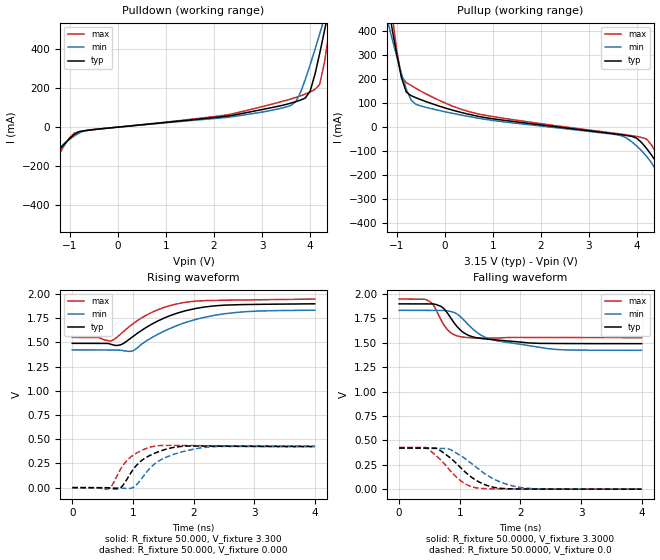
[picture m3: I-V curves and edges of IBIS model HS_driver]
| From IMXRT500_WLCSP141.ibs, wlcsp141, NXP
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[Model] HS_driver
|   Model HS_driver
| Library cells for typ/min/max conditions are connected as defined below:
|  pad_usbdp - External Pad
|  usb2_tx_d_data_dp - Core Input
|  gnda - gnda
|  pad_usb_vss - pad_usb_vss
|  usb2_reg_tx_fs_hiz - gnda
|  usb2_reg_tx_hs_term - vddd
|  usb2_reg_tx_hs_xcvr - vddd
|  usb2_reg_tx_ls_en - gnda
|  usbphy_d2a_txhsactive - vddd
|  vddb - vddb
|  vddd - vddd
| All other pins connected to ground
Model_type Output
Polarity   Non-Inverting
Enable   Active-High
C_comp   2.8431pF   2.6338pF   3.0727pF
[Temperature Range]   27.0000   0.1250k   -40.0000
[Voltage Range]   3.1500V   3.0000V   3.3000V
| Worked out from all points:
|   slope of the pulldown table from 0 to 0.472 V, typ, clamps not added: 41.5 ohm
|   slope of the pullup table from 0 to 0.472 V, typ, clamps not added: 18.7 ohm
|   rising waveform, R_fixture 50.000, V_fixture 3.300: 20-80 % time 788ps typ, 925ps min, 673ps max; typ from 1.49 V to 1.9 V
|   rising waveform, R_fixture 50.000, V_fixture 0.000: 20-80 % time 403ps typ, 514ps min, 316ps max; typ from 0 V to 0.424 V
|   falling waveform, R_fixture 50.0000, V_fixture 3.3000: 20-80 % time 376ps typ, 729ps min, 219ps max; typ from 1.9 V to 1.49 V
|   falling waveform, R_fixture 50.0000, V_fixture 0.0: 20-80 % time 478ps typ, 592ps min, 401ps max; typ from 0.422 V to 0 V
[Pulldown]
|Voltage   I(typ)   I(min)   I(max)
-3.3V     -1.789A    -1.328A    -2.415A
-2.1V     -625.7mA   -518.6mA   -789mA
-1.9V     -460.2mA   -400.2mA   -566.6mA
-1.4V     -174.1mA   -160.8mA   -216.9mA
-800mV    -22.89mA   -29.67mA   -23.37mA
3.6V      122.9mA    110.8mA    144.1mA
4V        183mA      317.7mA    180.5mA
4.2V      376.9mA    477.2mA    219mA
4.3V      493.6mA    559.9mA    332.1mA
4.4V      614.7mA    643.7mA    494.7mA
4.5V      738.7mA    728.1mA    671.8mA
6.6V      3.53A      2.592A     4.822A
[Pullup]
|Voltage   I(typ)   I(min)   I(max)
-3.3V     3.3A       2.299A     4.797A
-1.2V     532mA      451.2mA    654.1mA
-1.1V     415.8mA    372.2mA    481.1mA
-900mV    206.9mA    223.2mA    210.7mA
-700mV    130.9mA    112.5mA    173.3mA
700mV     45.05mA    37.34mA    54.91mA
3.9V      -38.79mA   -62.16mA   -35.71mA
4.3V      -115.3mA   -147.1mA   -73.13mA
4.6V      -211.6mA   -260.7mA   -191.1mA
4.9V      -368.9mA   -418mA     -342.3mA
5V        -440.4mA   -476.1mA   -413.1mA
6.6V      -1.963A    -1.562A    -2.435A
[Ramp]
| variable   typ   min   max
dV/dt_r  0.2425/0.3998n   0.2407/0.5102n   0.2458/0.3124n
dV/dt_f  0.2330/0.3629n   0.2298/0.6151n   0.2278/0.2332n
R_load = 45.0000
[Rising Waveform]
R_fixture = 50.000
V_fixture = 3.300
V_fixture_min = 3.000
V_fixture_max = 3.600
|  time   V(typ)   V(min)   V(max)
0s        1.489V     1.421V     1.55V
423.1ps   1.489V     1.421V     1.55V
635.7ps   1.48V      1.421V     1.514V
795.1ps   1.474V     1.417V     1.584V
989.5ps   1.554V     1.41V      1.686V
1.408ns   1.719V     1.581V     1.835V
1.906ns   1.831V     1.712V     1.917V
2.327ns   1.875V     1.776V     1.932V
2.7ns     1.887V     1.808V     1.936V
4ns       1.897V     1.831V     1.946V
[Rising Waveform]
R_fixture = 50.000
V_fixture = 0.000
V_fixture_min = 0.000
V_fixture_max = 0.000
|  time   V(typ)   V(min)   V(max)
0s        86.47nV    2.71uV     53.59nV
593.9ps   -1.371mV   1.709uV    -11.79mV
661ps     -10.2mV    -1.193uV   29.57mV
778.4ps   -6.653mV   -1.53mV    170.1mV
1.026ns   205.5mV    10.32mV    343.6mV
1.178ns   295.4mV    122.6mV    393.9mV
1.393ns   363.7mV    260.8mV    431.3mV
1.77ns    424.3mV    362.1mV    434.8mV
2.208ns   428.6mV    416.8mV    432.5mV
4ns       424.4mV    422.1mV    429.5mV
[Falling Waveform]
R_fixture= 50.0000
V_fixture= 3.3000
V_fixture_min= 3.0000
V_fixture_max= 3.6000
|time   V(typ)   V(min)   V(max)
0s        1.897V     1.831V     1.946V
504ps     1.897V     1.831V     1.921V
571.5ps   1.896V     1.831V     1.878V
686ps     1.872V     1.831V     1.738V
797.4ps   1.802V     1.826V     1.633V
1.027ns   1.62V      1.758V     1.559V
1.329ns   1.545V     1.585V     1.547V
1.664ns   1.526V     1.514V     1.549V
2.591ns   1.491V     1.431V     1.552V
4ns       1.49V      1.422V     1.551V
[Falling Waveform]
R_fixture= 50.0000
V_fixture= 0.0
V_fixture_min= 0.0
V_fixture_max= 0.0
|time   V(typ)   V(min)   V(max)
0s        421.7mV    418.5mV    427.2mV
441.6ps   421.8mV    418.5mV    426.2mV
625.8ps   415.8mV    418.5mV    335.7mV
805.8ps   339.1mV    414.1mV    216.4mV
994.4ps   232.6mV    351.5mV    95.97mV
1.262ns   93.77mV    228.8mV    14.73mV
1.448ns   38.4mV     144.5mV    4.904mV
1.624ns   12.57mV    85.57mV    2.638mV
2.041ns   1.956mV    14.67mV    1.342mV
4ns       435.6uV    536.4uV    364.7uV
